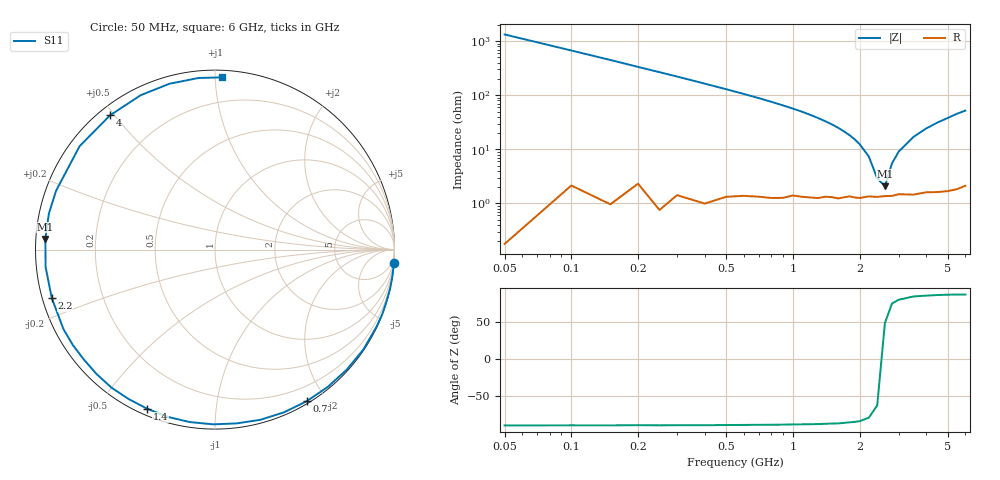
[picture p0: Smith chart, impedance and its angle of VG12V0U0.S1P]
! Infineon Technologies  Discrete & RF Semiconductors
! BB 831
! Si Tuning Diode in SOD323
! VR = 12 V
! S-Parameters:  July  1999
# GHz  S  MA  R  50
!  f  S11
! GHz  MAG  ANG
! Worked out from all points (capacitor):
!   34 points, 50 MHz to 6 GHz, reference 50 ohm
!   read as one part to ground: C = 2.36 pF near 50 MHz
!   lowest |Z| = 2.08 ohm at 2.6 GHz (marker M1)
!   series resonance near 2.524 GHz, so ESL is about 1.7 nH
!   S11 on the Smith chart (normalised r, x): 50 MHz: 0, -27; 700 MHz: 0.03, -1.77; 1.4 GHz: 0.03, -0.66; 2.2 GHz: 0.03, -0.14; 4 GHz: 0.03, +0.49; 6 GHz: 0.04, +1.04
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0.05  1 -4.3
0.15  0.9995 -12.7
0.25  0.999 -21.2
0.4  0.9966 -33.9
0.5  0.9931 -42.3
0.6  0.99 -50.6
0.7  0.9873 -58.8
0.8  0.9848 -67.0
0.9  0.9814 -75.1
1.1  0.9736 -90.6
1.2  0.9711 -98.3
1.3  0.9686 -105.8
1.4  0.9637 -113.1
1.6  0.9613 -126.9
1.7  0.9571 -133.7
1.9  0.954 -146.1
2  0.9537 -152.2
2.2  0.9486 -163.5
2.4  0.9488 -174.1
2.6  0.947 176.4
2.8  0.947 167.8
3  0.9443 159.7
3.5  0.9492 142.6
4  0.9495 128.0
4.5  0.9546 115.7
5  0.9582 105.4
5.5  0.9606 95.5
6  0.9602 87.7
